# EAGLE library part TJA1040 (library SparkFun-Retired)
CAN Tranceiver Retired
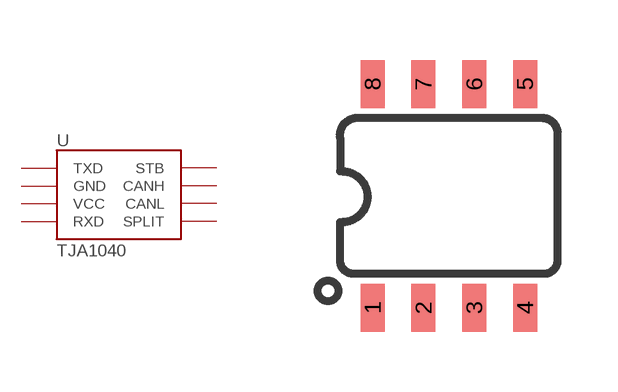
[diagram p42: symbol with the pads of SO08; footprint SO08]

Designator prefix -

## TJA1040  [SO08]
1  TXD
2  GND
3  VCC
4  RXD
5  SPLIT
6  CANL
7  CANH
8  STB

## Footprint SO08 (pad centres in mm)
SOIC, 0.15 inch width
smd 0.6 x 1.2: 1 -1.905,-2.8; 2 -0.635,-2.8; 3 0.635,-2.8; 4 1.905,-2.8; 5 1.905,2.8; 6 0.635,2.8; 7 -0.635,2.8; 8 -1.905,2.8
